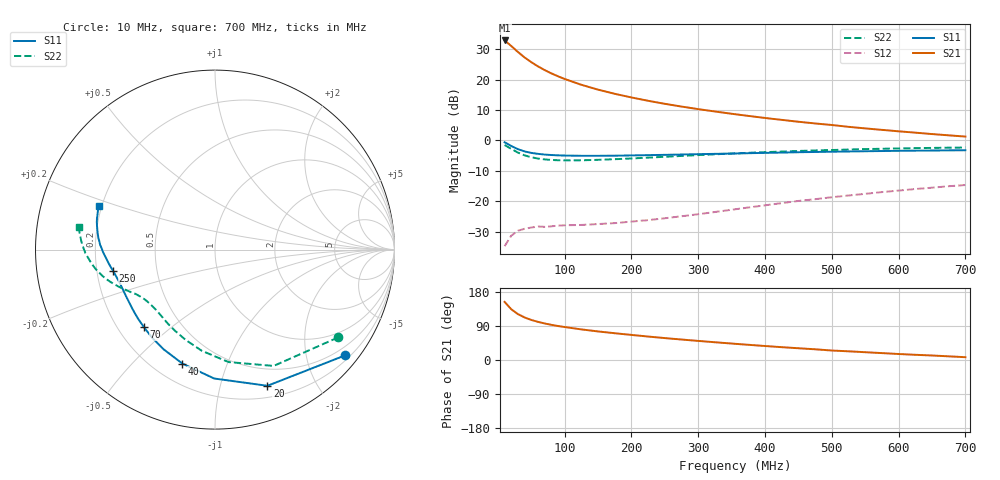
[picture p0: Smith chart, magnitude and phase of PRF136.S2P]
! Date: Mon Jul 31 13:38:03 1995
# MHZ  S  MA  R  50.0000
!  POLYFET RF DEVICES
!  PRF136
!  S PARAMETERS
!  VDS=28V, IDQ=200mA
!FREQ  S11MAG S11ANG S21MAG S21ANG S12MAG S12ANG S22MAG S22ANG
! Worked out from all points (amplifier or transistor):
!   34 points, 10 MHz to 700 MHz, reference 50 ohm
!   highest |S21| = 33.0 dB at 10 MHz (marker M1)
!   |S21| within 3 dB of that: start of sweep to 25.91 MHz
!   unconditionally stable (mu >= 1): 174.5 MHz to 381.2 MHz
!   at 60 MHz: K = 0.40, MSG = 26.4 dB, |S12| = -28.3 dB
!   at 300 MHz: K = 1.12, MAG = 15.2 dB, |S12| = -24.3 dB
!   at 700 MHz: K = 0.64, MSG = 8.0 dB, |S12| = -14.7 dB
!   S11 on the Smith chart (normalised r, x): 10 MHz: 0.30, -2.79; 20 MHz: 0.31, -1.41; 40 MHz: 0.31, -0.71; 70 MHz: 0.31, -0.40; 250 MHz: 0.27, -0.10; 700 MHz: 0.19, +0.17
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10  0.9347 -39.1  44.42 153.3  0.01817 68.6  0.8423 -35.5
20  0.813 -69.0  35.99 133.9  0.02707 51.0  0.7258 -63.2
30  0.7182 -90.4  28.65 121.0  0.03264 41.2  0.6311 -83.1
40  0.6602 -106.0  23.31 112.2  0.03513 35.7  0.5685 -97.4
50  0.6248 -117.4  19.47 105.7  0.03687 32.4  0.529 -108.0
60  0.6023 -125.8  16.61 100.6  0.03826 31.0  0.504 -116.3
70  0.5861 -132.5  14.45 96.4  0.03783 29.6  0.489 -122.5
80  0.5765 -137.9  12.74 92.8  0.03861 29.3  0.4779 -127.5
90  0.5693 -142.1  11.41 89.7  0.03958 30.1  0.4726 -131.2
100  0.5646 -145.6  10.3 87.0  0.04014 29.9  0.4699 -134.6
125  0.5597 -152.2  8.261 80.8  0.04064 32.6  0.4717 -140.6
150  0.5595 -157.0  6.876 75.4  0.04203 36.9  0.4805 -144.9
175  0.5617 -160.6  5.872 70.7  0.04355 40.4  0.4919 -147.9
200  0.5678 -163.6  5.11 66.2  0.04616 44.0  0.5055 -150.6
225  0.5737 -166.1  4.506 61.9  0.0488 48.8  0.5221 -152.8
250  0.5801 -168.2  4.018 57.8  0.05239 52.2  0.539 -154.9
300  0.5951 -172.1  3.285 50.4  0.06106 58.2  0.5751 -159.0
375  0.6176 -177.4  2.539 40.1  0.07877 63.5  0.6268 -164.7
425  0.632 179.3  2.185 33.8  0.09308 64.7  0.6573 -168.7
475  0.6469 175.7  1.908 28.3  0.1079 64.7  0.686 -172.6
600  0.6759 166.9  1.417 15.8  0.1495 60.9  0.7403 177.8
700  0.6908 159.6  1.161 7.4  0.1846 55.7  0.7651 170.7
